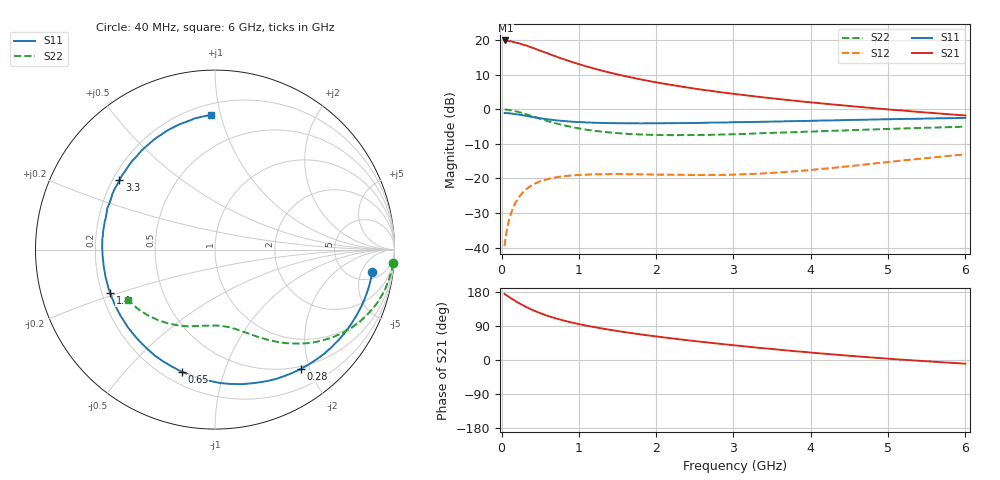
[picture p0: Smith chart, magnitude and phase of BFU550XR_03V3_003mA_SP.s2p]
! Filename:  P:\Prog\Test\Noise\ATS_data\Testdata_Net\03 Spar\BFU550XR_APG2013_45_C05_03p3V_003mA_SP_CM01_D.s2p
! Date/Time: Tue 06/Aug/2013 14:38:14
! BFU550XR_APG2013_45_C05_03p3V_1to35mA_SP_CM01_Bias3_R.s2p
! MDIF S-parameter v. bias file
! BFU550XR_APG2013_45_C05_03p3V_1to35mA_SP_CM01
! Date/time Fri Aug 02 14:41:13 2013
! VAR V_out= 3.3010
! VAR I_out= 3.0050
! VAR V_in= 0.8043
! VAR I_in= 0.0332
! Device data file deembeded for feedlines and parallel
! Original file: \03 Spar\BFU550XR_APG2013_45_C05_03p3V_003mA_SP_CM01_R.s2p
! Feed-files: PR006V01_02082013_Feed1.s2p, PR006V01_02082013_Feed2.s2p
! Parallel-file: PR006V01_02082013_Par.s2p
# MHz S MA R 50
!  Freq-MHz  S11-mag  S11-arg  S21-mag  S21-arg  S12-mag  S12-arg  S22-mag  S22-arg
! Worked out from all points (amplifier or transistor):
!   98 points, 40 MHz to 6 GHz, reference 50 ohm
!   highest |S21| = 19.9 dB at 50 MHz (marker M1)
!   |S21| within 3 dB of that: start of sweep to 506.5 MHz
!   unconditionally stable (mu >= 1): 2.758 GHz to 4.619 GHz
!   at 300 MHz: K = 0.13, MSG = 21.1 dB, |S12| = -23.5 dB
!   at 1.6 GHz: K = 0.61, MSG = 14.2 dB, |S12| = -18.8 dB
!   at 6 GHz: K = 0.84, MSG = 5.6 dB, |S12| = -13.0 dB
!   S11 on the Smith chart (normalised r, x): 40 MHz: 7, -8; 280 MHz: 0.46, -1.87; 650 MHz: 0.27, -0.73; 1.4 GHz: 0.23, -0.19; 3.3 GHz: 0.23, +0.31; 6 GHz: 0.27, +0.93
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40  0.886 -8.3  9.919 174.5  0.01046 85.1  0.9941 -4.4
50  0.8839 -10.3  9.925 172.3  0.01307 84.4  0.9936 -5.7
120  0.8703 -24.6  9.661 163.2  0.03049 75.9  0.9707 -13.9
180  0.8533 -36.2  9.272 155.7  0.04419 69.4  0.9395 -20.4
240  0.8326 -47.4  8.941 148.5  0.05619 63.6  0.9029 -26.2
280  0.8191 -54.2  8.594 144.2  0.06333 60.0  0.8762 -29.9
320  0.8032 -61.4  8.395 139.8  0.06963 56.5  0.8476 -33.3
440  0.7618 -79.7  7.499 128.6  0.08494 48.0  0.7678 -41.9
550  0.7287 -94.2  6.754 119.8  0.09447 41.5  0.7004 -48.4
650  0.7055 -105.2  6.118 113.1  0.1011 37.0  0.6516 -53.0
750  0.6863 -115.0  5.571 107.1  0.1056 33.3  0.6086 -57.1
850  0.6705 -123.8  5.105 101.8  0.109 30.1  0.5723 -60.6
1050  0.6502 -138.2  4.337 92.7  0.1127 25.4  0.5174 -66.5
1400  0.6315 -157.4  3.403 79.8  0.1153 20.4  0.4624 -74.5
1700  0.6269 -170.2  2.861 70.5  0.1148 18.3  0.4371 -80.4
2050  0.6288 177.7  2.403 60.9  0.1135 17.8  0.4246 -86.7
2500  0.6334 164.2  1.993 49.9  0.1123 19.1  0.4254 -94.3
3100  0.6534 148.7  1.627 36.9  0.1147 24.4  0.4394 -104.0
3300  0.6576 144.1  1.528 32.8  0.1168 26.2  0.4487 -107.3
4100  0.6865 126.9  1.231 17.9  0.136 33.0  0.4804 -120.3
5200  0.7259 105.7  0.9572 0.6  0.1826 35.1  0.5284 -137.7
6000  0.7511 91.9  0.8149 -9.7  0.2229 31.7  0.5608 -150.1
